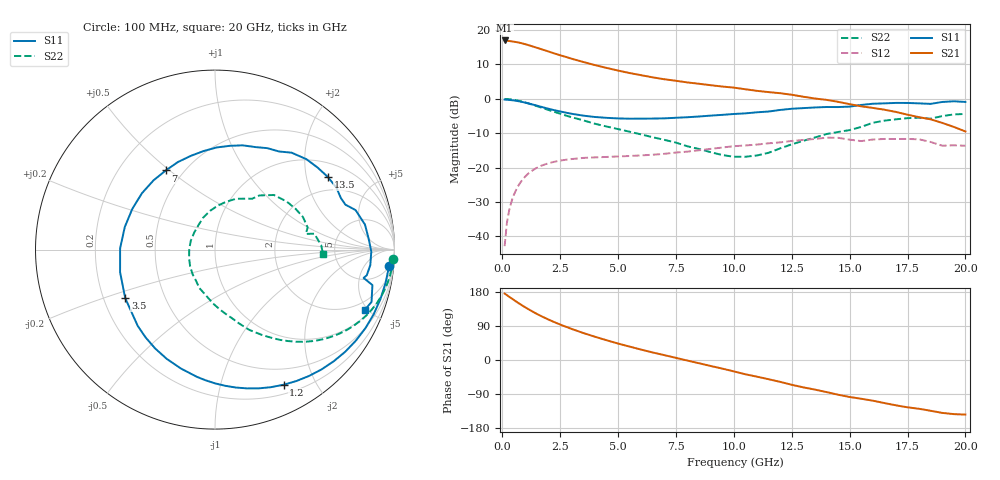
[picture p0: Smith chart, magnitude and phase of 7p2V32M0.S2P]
! Infineon Technologies  Discrete & RF Semiconductors
! bfp620
! VCE =  2.3 V,  IC =  2.0 mA
! Common Emitter S-Parameters:  Sep 2002
# GHz  S  MA  R  50
!  f  S11  S21  S12  S22
! GHz  MAG  ANG  MAG  ANG  MAG  ANG  MAG  ANG
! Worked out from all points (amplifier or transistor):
!   59 points, 100 MHz to 20 GHz, reference 50 ohm
!   highest |S21| = 17.0 dB at 100 MHz (marker M1)
!   |S21| within 3 dB of that: start of sweep to 1.897 GHz
!   unconditionally stable (mu >= 1): 5.735 GHz to 13.97 GHz; 14.02 GHz to 15.62 GHz; 17.66 GHz to end of sweep
!   at 1 GHz: K = 0.16, MSG = 19.2 dB, |S12| = -22.5 dB
!   at 5.5 GHz: K = 0.97, MSG = 12.1 dB, |S12| = -16.6 dB
!   at 20 GHz: K = 1.30, MAG = -1.2 dB, |S12| = -13.7 dB
!   S11 on the Smith chart (normalised r, x): 100 MHz: 5, -20; 1.2 GHz: 0.30, -1.59; 3.5 GHz: 0.29, -0.23; 7 GHz: 0.40, +0.48; 13.5 GHz: 1.46, +2.68; 20 GHz: 1.36, -4.80
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0.1  0.9744 -5.4  7.045 175.2  0.0072 81.9  0.9947 -3.1
0.2  0.9684 -11.0  6.977 171.1  0.0158 81.3  0.9908 -6.2
0.3  0.9622 -16.6  6.912 166.8  0.0241 79.3  0.9843 -9.3
0.7  0.9222 -38.1  6.573 150.2  0.055 67.7  0.9351 -21.0
0.9  0.8932 -48.4  6.333 142.4  0.0685 61.7  0.9002 -26.3
1.2  0.8443 -63.1  5.924 131.5  0.0858 53.1  0.8413 -33.5
1.4  0.8105 -72.5  5.645 124.7  0.0954 48.0  0.8007 -37.8
1.7  0.761 -85.7  5.241 115.3  0.1068 41.1  0.7415 -43.5
2.2  0.689 -106.1  4.62 101.2  0.1204 31.6  0.6532 -51.3
2.8  0.6231 -128.5  4.008 86.6  0.1306 22.7  0.5632 -59.2
3.5  0.5686 -151.6  3.426 71.2  0.1382 14.5  0.4853 -67.0
4  0.5437 -166.6  3.089 61.4  0.1406 9.6  0.4339 -71.8
5  0.5182 165.9  2.571 43.4  0.1451 3.1  0.3628 -80.6
6  0.5142 142.3  2.201 27.4  0.1503 -1.7  0.3032 -91.4
7  0.5193 121.9  1.923 12.8  0.1584 -5.3  0.2529 -103.4
9  0.5691 89.1  1.576 -15.8  0.1869 -14.9  0.1674 -145.8
10.5  0.6139 68.5  1.375 -37.7  0.2096 -25.8  0.1437 160.2
12  0.6882 51.7  1.205 -57.7  0.2326 -35.6  0.1902 110.1
13.5  0.7477 32.8  1.009 -78.1  0.2606 -49.1  0.2735 76.9
15  0.7687 19.0  0.836 -97.6  0.2545 -68.4  0.3508 53.9
17  0.8708 -0.7  0.644 -119.6  0.2602 -81.3  0.503 26.9
20  0.8998 -21.9  0.335 -144.1  0.2075 -103.3  0.6027 -2.5
